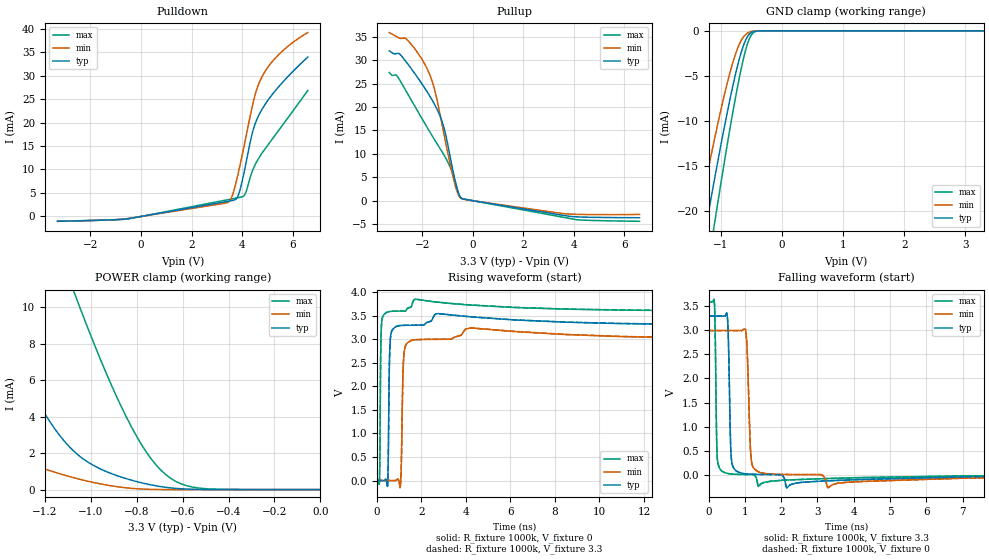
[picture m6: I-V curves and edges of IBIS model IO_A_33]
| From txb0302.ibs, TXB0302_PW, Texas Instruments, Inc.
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[Model]   IO_A_33
Model_type  3-state
Enable   Active-High
Vref =   0
Rref =   1000K
Cref =   50p
Vmeas =   1.65
| variable   typ   min   max
C_comp   3.23pF   2.99pF   3.44pF
| C_pullup   3.42pF   3.11pF   3.58pF
| C_pulldown   3.42pF   3.11pF   3.58pF
| C_tri-state   3.23pF   2.99pF   3.44pF
[Temperature Range]   40   100   -40
| Ambient temperature   25   85   -40
[Voltage range]   3.3   3   3.6
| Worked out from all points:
|   slope of the pulldown table from 0 to 0.495 V, typ, clamps not added: 1.07 kohm
|   slope of the pullup table from 0 to 0.495 V, typ, clamps not added: 1.14 kohm
|   GND clamp passes 1 mA (typ) near -0.59 V on its own axis
|   POWER clamp passes 1 mA (typ) near -0.93 V on its own axis
|   rising waveform, R_fixture 1000k, V_fixture 0: 20-80 % time 54.5ps typ, 74.1ps min, 38.6ps max; typ from 0 V to 3.3 V
|   falling waveform, R_fixture 1000k, V_fixture 3.3: 20-80 % time 54.5ps typ, 76.5ps min, 39ps max; typ from 3.3 V to 0.004 V
|   rising waveform, R_fixture 1000k, V_fixture 3.3: 20-80 % time 54.7ps typ, 74.4ps min, 38.7ps max; typ from 0.004 V to 3.3 V
|   falling waveform, R_fixture 1000k, V_fixture 0: 20-80 % time 54.6ps typ, 76.6ps min, 39ps max; typ from 3.3 V to 0 V
[GND Clamp]
| IO_A_33
|   Voltage   I(typ)   I(min)   I(max)
-3.3V     -107.8mA   -94.82mA   -123.5mA
-1.4V     -27.92mA   -22.08mA   -34.6mA
-1.355V   -26.16mA   -20.51mA   -32.58mA
-1.24V    -21.7mA    -16.57mA   -27.47mA
-1.105V   -16.6mA    -12.13mA   -21.56mA
-930mV    -10.32mA   -6.816mA   -14.13mA
-780mV    -5.448mA   -3.031mA   -8.201mA
-650mV    -2.065mA   -895.1uA   -3.734mA
-540mV    -437.9uA   -178.1uA   -1.021mA
-465mV    -87.77uA   -39.15uA   -208.4uA
-365mV    -6.098uA   -3.222uA   -9.086uA
3.3V      878.5pA    29.7nA     71.4pA
[POWER Clamp]
| IO_A_33
|   Voltage   I(typ)   I(min)   I(max)
-3.3V     75.76mA    55.16mA    102.1mA
-1.87V    23.53mA    10.79mA    41.25mA
-1.62V    15.48mA    5.161mA    31.23mA
-1.465V   10.85mA    2.838mA    25.17mA
-1.225V   4.661mA    1.234mA    16.15mA
-1.065V   1.999mA    620.1uA    10.55mA
-935mV    1mA        257uA      6.436mA
-830mV    541.2uA    77.16uA    3.598mA
-740mV    263.8uA    13.45uA    1.73mA
-670mV    119.9uA    2.07uA     782.6uA
-510mV    6.607uA    44.4nA     59.35uA
0V        0A         0A         0A
[Pulldown]
| IO_A_33
|   Voltage   I(typ)   I(min)   I(max)
-3.3V     -1.028mA   -1.023mA   -1.025mA
-535mV    -493.8uA   -452.8uA   -534.3uA
3.47V     3.253mA    3.116mA    3.608mA
3.64V     3.422mA    4.863mA    3.785mA
3.865V    4.743mA    9.657mA    4.019mA
4.12V     10.46mA    16.1mA     4.792mA
4.415V    17.96mA    23.74mA    9.781mA
4.565V    20.4mA     26.8mA     11.51mA
4.735V    22.3mA     29.17mA    13.04mA
5.03V     24.79mA    31.85mA    15.28mA
5.445V    27.6mA     34.44mA    18.31mA
6.6V      33.95mA    39.15mA    26.82mA
[Pullup]
| IO_A_33
|   Voltage   I(typ)   I(min)   I(max)
-3.3V     32.02mA    35.91mA    27.37mA
-3V       31.45mA    35.01mA    26.69mA
-2.58V    29.27mA    34.29mA    22.89mA
-2.095V   25.64mA    30.93mA    18.34mA
-1.74V    22.71mA    27.43mA    15.08mA
-1.485V   20.31mA    23.24mA    12.81mA
-1.18V    16.39mA    15.37mA    10.15mA
-715mV    4.751mA    3.73mA     4.54mA
-580mV    1.881mA    1.434mA    1.907mA
-465mV    627.7uA    529.4uA    613uA
4.11V     -3.458mA   -2.919mA   -4.054mA
6.6V      -3.647mA   -2.946mA   -4.405mA
[Ramp]
| IO_A_33
| variable   typ   min   max
dV/dt_r   2.21/7.21E-11   2.04/9.96E-11   2.36/4.82E-11
dV/dt_f   2.18/6.74E-11   1.98/9.57E-11   2.34/4.59E-11
R_load = 1000k
[Rising Waveform]
| IO_A_33
R_fixture =   1000k
C_fixture =   0
L_fixture =   0
V_fixture =   0
V_fixture_min = 0
V_fixture_max = 0
|   Time   V(typ)   V(min)   V(max)
0s        734nV      3.093uV    102.7nV
125ps     -97.32uV   3.003uV    44.59mV
181ps     66.7uV     2.896uV    2.866V
245ps     -60.03uV   2.942uV    3.445V
485ps     -111.5mV   -30.3uV    3.579V
645ps     3.135V     16.9uV     3.592V
1.053ns   3.291V     -139mV     3.599V
1.229ns   3.296V     2.721V     3.596V
1.741ns   3.299V     2.991V     3.85V
37.68ns   3.296V     2.996V     3.596V
[Falling Waveform]
| IO_A_33
R_fixture =   1000k
C_fixture =   0
L_fixture =   0
V_fixture =   3.3
V_fixture_min = 3
V_fixture_max = 3.6
|   Time   V(typ)   V(min)   V(max)
0s        3.3V       3V         3.6V
165ps     3.3V       3V         3.539V
229ps     3.3V       3V         575.7mV
261ps     3.3V       3V         223.3mV
525ps     3.236V     3V         24.4mV
637ps     272mV      3V         11.83mV
1.021ns   15.18mV    3.023V     1.824mV
1.165ns   6.833mV    419.9mV    1.117mV
1.373ns   2.589mV    58.47mV    -249.3mV
37.68ns   3.586mV    3.893mV    3.47mV
[Rising Waveform]
| IO_A_33
R_fixture =   1000k
C_fixture =   0
L_fixture =   0
V_fixture =   3.3
V_fixture_min = 3
V_fixture_max = 3.6
|   Time   V(typ)   V(min)   V(max)
0s        3.501mV    3.512mV    3.456mV
125ps     3.403mV    3.512mV    48mV
181ps     3.567mV    3.511mV    2.868V
245ps     3.441mV    3.512mV    3.446V
485ps     -108mV     3.478mV    3.579V
645ps     3.135V     3.525mV    3.592V
1.053ns   3.291V     -135.6mV   3.599V
1.229ns   3.296V     2.721V     3.596V
1.741ns   3.299V     2.991V     3.852V
37.68ns   3.3V       3V         3.6V
[Falling Waveform]
| IO_A_33
R_fixture =   1000k
C_fixture =   0
L_fixture =   0
V_fixture =   0
V_fixture_min = 0
V_fixture_max = 0
|   Time   V(typ)   V(min)   V(max)
0s        3.296V     2.996V     3.596V
165ps     3.296V     2.996V     3.535V
229ps     3.296V     2.996V     574.2mV
261ps     3.296V     2.996V     223mV
525ps     3.233V     2.996V     24.31mV
637ps     271.4mV    2.996V     11.75mV
1.021ns   15.09mV    3.019V     1.752mV
1.165ns   6.757mV    418.6mV    1.046mV
1.373ns   2.517mV    58.33mV    -249.2mV
37.68ns   87.56uV    386.3uV    14.54uV
